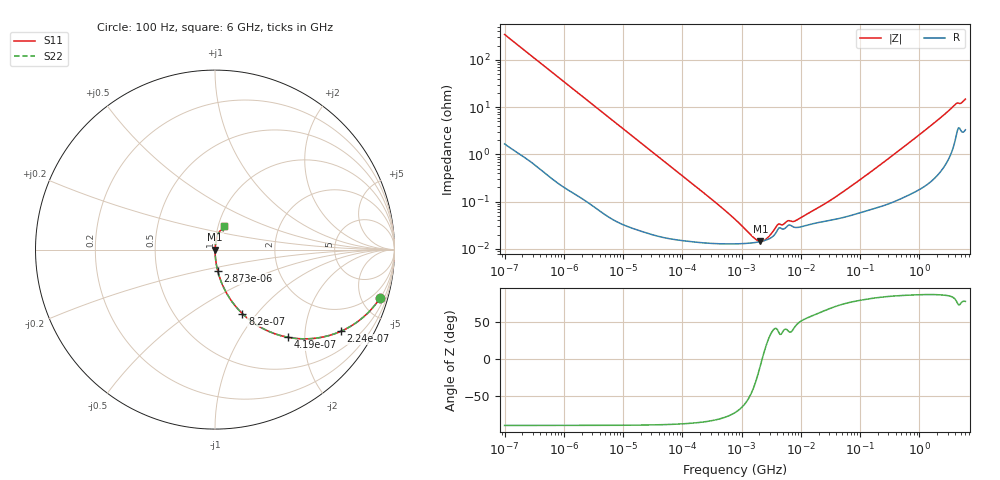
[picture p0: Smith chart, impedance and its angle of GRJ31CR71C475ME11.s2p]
!Murata Part Number: GRJ31CR71C475ME11
!These Parameters are Measured in Series Mode Connection
!Data Generated on Jun 19, 2026
!  o--ll--o
!Port1  Port2
!  o------o
!Operation Temp=25[degC], DC Bias Voltage=0[V]
!Freq. Start=100[Hz] Stop=6[GHz] 401[Steps]
# Hz S RI R 50
!Freq.(Hz) S11(Real) S11(Imag) S21(Real) S21(Imag) S12(Real) S12(Imag) S22(Real) S22(Imag)
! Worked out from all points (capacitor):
!   401 points, 100 Hz to 6 GHz, reference 50 ohm
!   read as one part in series: C = 4.62 uF near 109 Hz
!   lowest |Z| = 14.5 mohm at 2.074 MHz (marker M1)
!   series resonance near 2.234 MHz, so ESL is about 1.1 nH
!   S11 on the Smith chart (normalised r, x): 100 Hz: 1.03, -6.88; 224 Hz: 1.02, -3.08; 419 Hz: 1.01, -1.65; 820 Hz: 1.00, -0.84; 2.873 kHz: 1.00, -0.24; 6 GHz: 1.07, +0.29
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100  0.921 -0.2673  0.079 0.2673  0.079 0.2673  0.921 -0.2673
150  0.84 -0.3641  0.16 0.3641  0.16 0.3641  0.84 -0.3641
224  0.7026 -0.4544  0.2974 0.4544  0.2974 0.4544  0.7026 -0.4544
419  0.4056 -0.4882  0.5944 0.4882  0.5944 0.4882  0.4056 -0.4882
820  0.1528 -0.357  0.8472 0.357  0.8472 0.357  0.1528 -0.357
2008  0.0301 -0.1677  0.9699 0.1677  0.9699 0.1677  0.0301 -0.1677
2873  0.0153 -0.1192  0.9847 0.1192  0.9847 0.1192  0.0153 -0.1192
8416  0.00208 -0.0414  0.9979 0.0414  0.9979 0.0414  0.00208 -0.0414
40335  0.000259 -0.00871  0.9997 0.00871  0.9997 0.00871  0.000259 -0.00871
774597  0.000128 -0.000405  0.9999 0.000405  0.9999 0.000405  0.000128 -0.000405
1585629  0.000135 -0.000112  0.9999 0.000112  0.9999 0.000112  0.000135 -0.000112
2074311  0.000143 -2.38e-05  0.9999 2.38e-05  0.9999 2.38e-05  0.000143 -2.38e-05
2713602  0.000157 6.4e-05  0.9998 -6.4e-05  0.9998 -6.4e-05  0.000157 6.4e-05
4060267  0.000254 0.000202  0.9997 -0.000202  0.9997 -0.000202  0.000254 0.000202
6075234  0.000312 0.000241  0.9997 -0.000241  0.9997 -0.000241  0.000312 0.000241
7947587  0.000285 0.000265  0.9997 -0.000265  0.9997 -0.000265  0.000285 0.000265
1.555665e7  0.000338 0.000534  0.9997 -0.000534  0.9997 -0.000534  0.000338 0.000534
4.764863e7  0.000452 0.00144  0.9995 -0.00144  0.9995 -0.00144  0.000452 0.00144
3.124326e8  0.000979 0.00837  0.999 -0.00837  0.999 -0.00837  0.000979 0.00837
1.497423e9  0.004 0.0384  0.996 -0.0384  0.996 -0.0384  0.004 0.0384
4.009986e9  0.0305 0.1057  0.9695 -0.1057  0.9695 -0.1057  0.0305 0.1057
6e9  0.0504 0.1322  0.9496 -0.1322  0.9496 -0.1322  0.0504 0.1322
